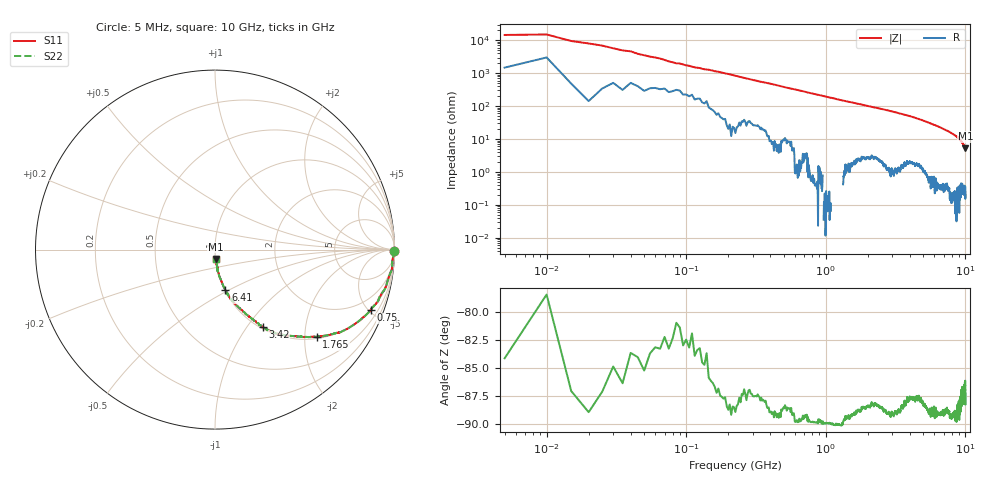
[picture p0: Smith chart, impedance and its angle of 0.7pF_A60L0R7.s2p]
! Amotech Co.,Ltd.
! http://www.amotech.co.kr/
! Part Number: A60L0R7
! These Parameters are Measured in Series Mode Connection
! Operation Temp=25[degC], DC Bias Voltage=0[V]
! Freq. Start=5[MHz] Stop=10[GHz], 2000[Steps]
! Date: Monday, July 14, 2020, 09:26:33
# GHZ S RI R 50.000000
!Freq.(Hz) S11(Real) S11(Imag) S21(Real) S21(Imag) S12(Real) S12(Imag) S22(Real) S22(Imag)
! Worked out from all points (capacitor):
!   2000 points, 5 MHz to 10 GHz, reference 50 ohm
!   read as one part in series: C = 910 fF near 55 MHz
!   lowest |Z| = 5.22 ohm at 9.995 GHz (marker M1)
!   S11 on the Smith chart (normalised r, x): 5 MHz: open; 750 MHz: 1.01, -5.14; 1.765 GHz: 1.04, -2.29; 3.42 GHz: 1.02, -1.19; 6.41 GHz: 1.01, -0.48; 10 GHz: 1.01, -0.11
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0.005  0.9993 -0.00684  0.000748 0.00684  0.000748 0.00684  0.9993 -0.00684
0.03  0.9981 -0.0174  0.00186 0.0174  0.00186 0.0174  0.9981 -0.0174
0.07  0.9932 -0.0387  0.00681 0.0387  0.00681 0.0387  0.9932 -0.0387
0.095  0.9906 -0.0531  0.00944 0.0531  0.00944 0.0531  0.9906 -0.0531
0.135  0.9875 -0.0741  0.0125 0.0741  0.0125 0.0741  0.9875 -0.0741
0.21  0.9865 -0.1089  0.0135 0.1089  0.0135 0.1089  0.9865 -0.1089
0.305  0.968 -0.1561  0.032 0.1561  0.032 0.1561  0.968 -0.1561
0.42  0.9519 -0.2061  0.0481 0.2061  0.0481 0.2061  0.9519 -0.2061
0.75  0.8679 -0.3372  0.1321 0.3372  0.1321 0.3372  0.8679 -0.3372
1.21  0.7227 -0.4486  0.2773 0.4486  0.2773 0.4486  0.7227 -0.4486
1.675  0.5863 -0.4833  0.4137 0.4833  0.4137 0.4833  0.5863 -0.4833
1.765  0.5659 -0.4863  0.4341 0.4863  0.4341 0.4863  0.5659 -0.4863
2.51  0.4036 -0.4785  0.5964 0.4785  0.5964 0.4785  0.4036 -0.4785
3.34  0.2747 -0.4361  0.7253 0.4361  0.7253 0.4361  0.2747 -0.4361
3.42  0.2665 -0.432  0.7335 0.432  0.7335 0.432  0.2665 -0.432
5.005  0.1236 -0.3143  0.8764 0.3143  0.8764 0.3143  0.1236 -0.3143
6.41  0.0577 -0.2258  0.9423 0.2258  0.9423 0.2258  0.0577 -0.2258
6.67  0.0499 -0.2106  0.9501 0.2106  0.9501 0.2106  0.0499 -0.2106
8.335  0.019 -0.1313  0.981 0.1313  0.981 0.1313  0.019 -0.1313
9.24  0.01 -0.0902  0.99 0.0902  0.99 0.0902  0.01 -0.0902
9.995  0.00424 -0.0519  0.9958 0.0519  0.9958 0.0519  0.00424 -0.0519
10  0.00523 -0.0521  0.9948 0.0521  0.9948 0.0521  0.00523 -0.0521
